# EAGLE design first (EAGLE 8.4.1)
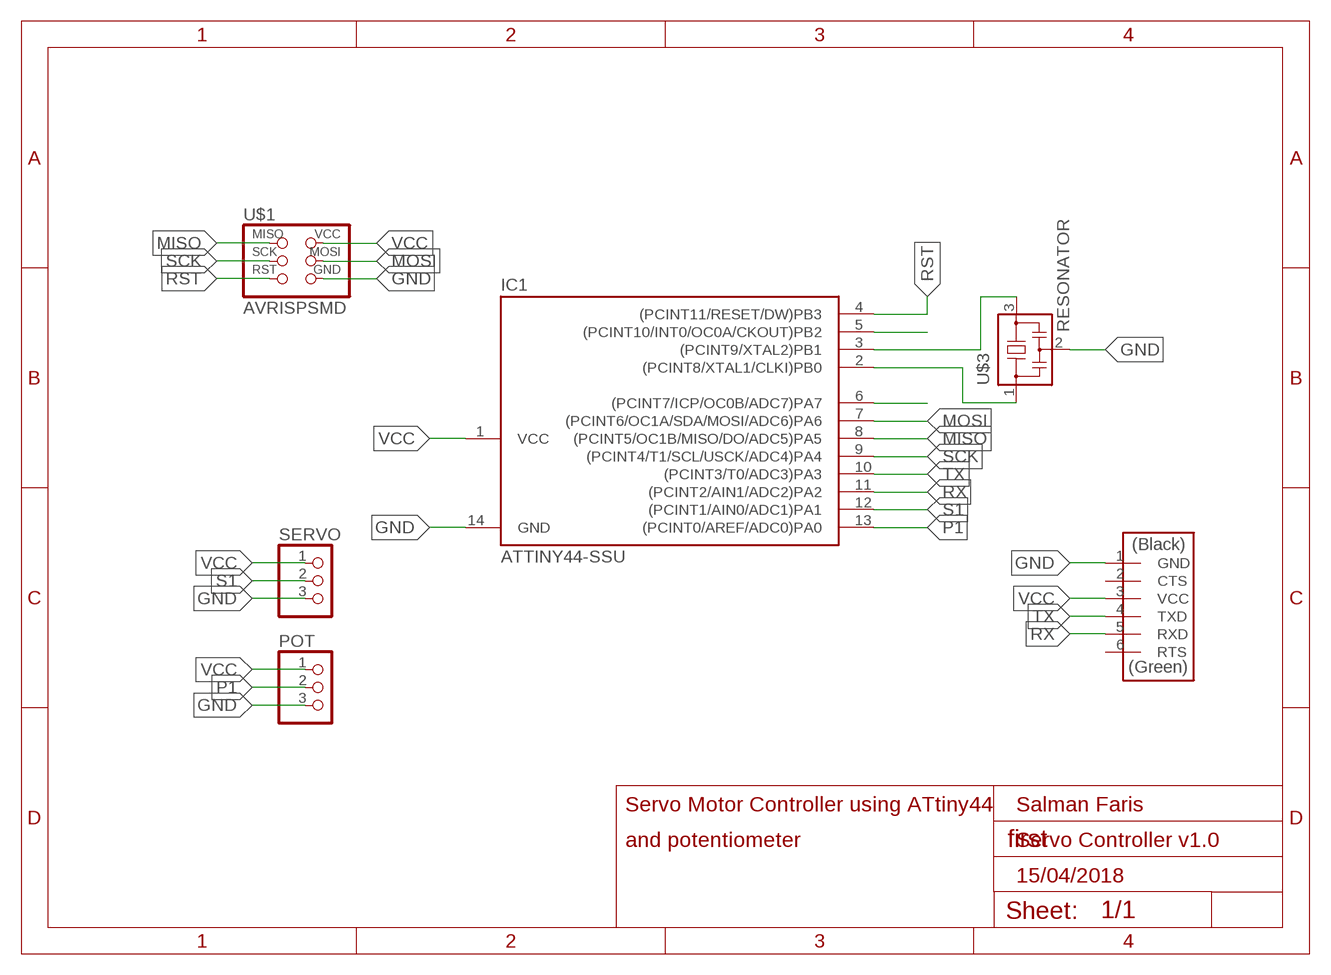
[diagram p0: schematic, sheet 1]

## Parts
IC1  ATTINY44-SSU  [SOIC14]
POT  PINHD-1X3  [1X03]
SERVO  PINHD-1X3  [1X03]
U$1  AVRISPSMD  [2X03SMD]
U$2  FTDI-SMD-HEADER  [1X06SMD]
U$3  RESONATOR  [EFOBM]

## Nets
GND: IC1.14(GND) POT.3 SERVO.3 U$1.6(GND) U$2.1(GND) U$3.2
MISO: IC1.8((PCINT5/OC1B/MISO/DO/ADC5)PA5) U$1.1(MISO)
MOSI: IC1.7((PCINT6/OC1A/SDA/MOSI/ADC6)PA6) U$1.4(MOSI)
N$10: IC1.5((PCINT10/INT0/OC0A/CKOUT)PB2)
N$11: IC1.3((PCINT9/XTAL2)PB1) U$3.3
N$12: IC1.2((PCINT8/XTAL1/CLKI)PB0) U$3.1
N$13: IC1.6((PCINT7/ICP/OC0B/ADC7)PA7)
P1: IC1.13((PCINT0/AREF/ADC0)PA0) POT.2
RST: IC1.4((PCINT11/RESET/DW)PB3) U$1.5(RST)
RX: IC1.11((PCINT2/AIN1/ADC2)PA2) U$2.5(RXD)
S1: IC1.12((PCINT1/AIN0/ADC1)PA1) SERVO.2
SCK: IC1.9((PCINT4/T1/SCL/USCK/ADC4)PA4) U$1.3(SCK)
TX: IC1.10((PCINT3/T0/ADC3)PA3) U$2.4(TXD)
VCC: IC1.1(VCC) POT.1 SERVO.1 U$1.2(VCC) U$2.3(VCC)
Unconnected: U$2.2(CTS) U$2.6(RTS)

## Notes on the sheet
- Servo Motor Controller using ATtiny44 | Salman Faris
- and potentiometer | Servo Controller v1.0
- 15/04/2018

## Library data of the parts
IC1 = fab:ATTINY44
POT SERVO = pinhead:PINHD-1X3: PIN HEADER
U$1 = fab:AVRISP
U$2 = fab:FTDI-SMD-HEADER
U$3 = fab:RESONATOR

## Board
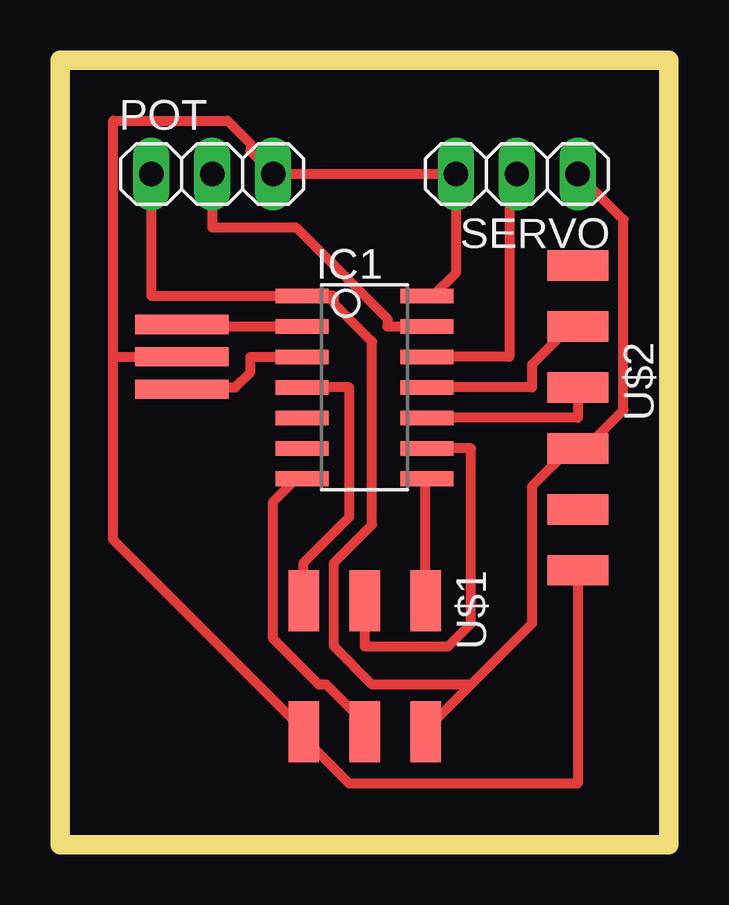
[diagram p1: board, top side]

Size 25.38 x 32.69 mm. Coordinates in mm from the lower left corner, seen from the top.
Outline: 0,0 25.38,0 25.38,32.69 0,32.69 0,0
Copper layers (1*16): Top 0.035mm / dielectric 1.5mm / Bottom 0.035mm
Design rules "default *": minimum track width 16mil, minimum drill 0.35mm, track to track 16mil, track to pad 16mil, pad to pad 16mil, via to via 16mil, smd to smd 16mil, copper to edge 16mil, drill to drill 16mil, minimum pad ring 10mil, minimum via ring 8mil, stop-mask expansion 4mil, vias tented up to drill 0mil, thermal gap 10mil

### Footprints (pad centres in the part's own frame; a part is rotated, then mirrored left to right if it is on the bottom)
SOIC14 = smd 0.61 x 2.21: 1 -3.81,-2.603; 2 -2.54,-2.603; 3 -1.27,-2.603; 4 0,-2.603; 5 1.27,-2.603; 6 2.54,-2.603; 7 3.81,-2.603; 8 3.81,2.603; 9 2.54,2.603; 10 1.27,2.603; 11 0,2.603; 12 -1.27,2.603; 13 -2.54,2.603; 14 -3.81,2.603
1X03 = drill 1.016 long: 1 -2.54,0; 2 0,0; 3 2.54,0
2X03SMD = smd 2.54 x 1.27: 1 -2.54,2.54; 2 2.92,2.54; 3 -2.54,0; 4 2.92,0; 5 -2.54,-2.54; 6 2.92,-2.54
1X06SMD = smd 2.54 x 1.27: 1 0,6.35; 2 0,3.81; 3 0,1.27; 4 0,-1.27; 5 0,-3.81; 6 0,-6.35
EFOBM = smd 0.8 x 3.9: 1 -1.35,0; 2 0,0; 3 1.35,0

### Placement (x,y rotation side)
IC1  12.7,19.05 270 top
POT  6.35,27.94 0 top
SERVO  19.05,27.94 180 top
U$1  12.7,7.62 270 top
U$2  21.59,17.78 180 top
U$3  5.08,20.32 270 top

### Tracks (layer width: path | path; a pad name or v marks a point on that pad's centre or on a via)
GND
  Top 0.406: IC1.14 15.56,22.86 16.51,23.81 SERVO.3 POT.3 7.94,28.89 7.94,29.21 6.99,30.16 2.22,30.16 2.22,20.32 | U$2.1 21.59,2.54 12.06,2.54 10.16,4.45 U$1.6 10.16,4.76 2.22,12.7 2.22,20.32 | 2.22,20.32 U$3.2
MISO
  Top 0.406: U$1.1 15.24,15.24 IC1.8
MOSI
  Top 0.406: U$1.4 12.7,5.08 11.11,6.67 10.79,6.67 8.89,8.57 8.89,14.29 9.84,15.24 IC1.7
N$11
  Top 0.406: IC1.3 7.94,20.32 7.94,19.68 7.3,19.05 5.08,19.05 U$3.3
N$12
  Top 0.406: IC1.2 5.08,21.59 U$3.1
P1
  Top 0.406: IC1.13 13.65,21.59 13.65,21.91 9.84,25.72 6.35,25.72 POT.2
RST
  Top 0.406: IC1.4 12.06,19.05 12.06,13.65 10.16,11.75 U$1.5
RX
  Top 0.406: IC1.11 19.68,19.05 19.68,20 21.27,21.59 U$2.5
S1
  Top 0.406: IC1.12 18.73,20.32 18.73,27.62 SERVO.2
SCK
  Top 0.406: IC1.9 17.14,16.51 17.14,9.21 16.19,8.26 12.7,8.26 U$1.3
TX
  Top 0.406: IC1.10 21.59,17.78 U$2.4
VCC
  Top 0.406: POT.1 3.81,22.86 IC1.1 11.43,22.86 11.43,22.54 13.02,20.96 13.02,13.34 11.43,11.75 11.43,8.26 13.02,6.67 17.14,6.67 | 17.14,6.67 19.68,9.21 19.68,14.92 21.27,16.51 U$2.3 21.91,16.51 23.5,18.1 23.5,26.04 SERVO.1 | 17.14,6.67 15.24,4.76 U$1.2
